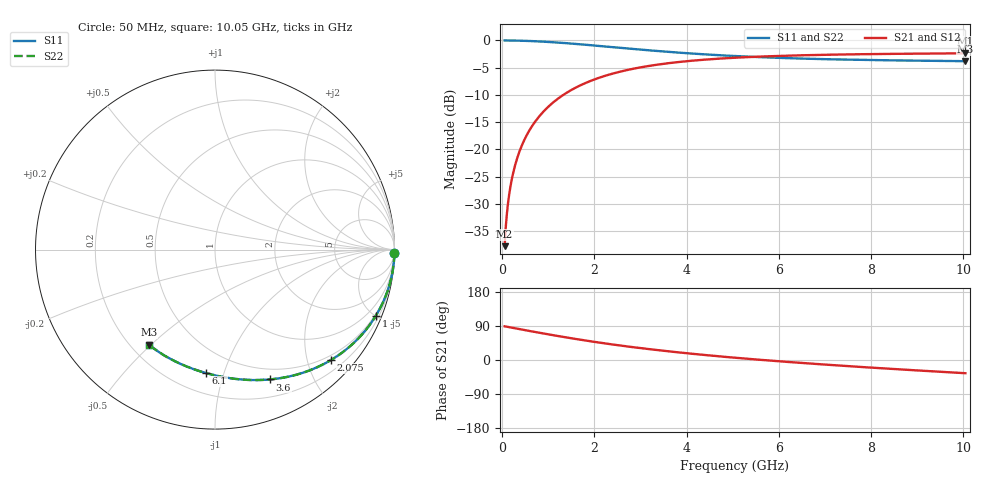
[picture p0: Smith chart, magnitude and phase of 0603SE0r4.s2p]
! AVX Thin Film Operation		Date: August 2001
! Description: Accu-P® Series, Thin Film, SMD, RF Capacitor
! Part Number: 06035J0R4ABT
! 50 MHz  -  10.05 GHz
! Serial Measurements
# mhz S db R 50
!	S11		S21		S12		S22
!	dB	Phase	dB	Phase	dB	Phase	dB	Phase
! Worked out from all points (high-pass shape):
!   401 points, 50 MHz to 10.05 GHz, reference 50 ohm
!   highest |S21| = -2.36 dB at 10.05 GHz (marker M1); lowest = -37.8 dB at 50 MHz (marker M2)
!   |S21| within 3 dB of the highest: 2.751 GHz to end of sweep
!   lowest |S11| = -3.8 dB at 10.05 GHz (marker M3), VSWR 4.64, Z = 13.6 - j24.6 ohm
!   |S11| at or under -10 dB: nowhere
!   |S22| runs from -3.8 to 0.0 dB; largest |S21 - S12| = 6.7e-05
!   S11 on the Smith chart (normalised r, x): 50 MHz: open; 1 GHz: 0.42, -5.02; 2.075 GHz: 0.41, -2.45; 3.6 GHz: 0.38, -1.44; 6.1 GHz: 0.33, -0.87; 10.05 GHz: 0.27, -0.49
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50  -0.00 -1.1  -37.79 88.9  -37.79 88.9  -0.00 -1.1
75  -0.00 -1.7  -34.27 88.3  -34.27 88.3  -0.00 -1.7
125  -0.00 -2.9  -29.84 87.1  -29.84 87.1  -0.00 -2.9
175  -0.01 -4.0  -26.92 86.0  -26.92 86.0  -0.01 -4.0
250  -0.02 -5.7  -23.84 84.3  -23.84 84.3  -0.02 -5.7
350  -0.04 -8.0  -20.94 82.0  -20.94 82.0  -0.04 -8.0
475  -0.07 -10.8  -18.33 79.2  -18.33 79.2  -0.07 -10.8
625  -0.11 -14.2  -16.01 75.8  -16.01 75.8  -0.11 -14.2
800  -0.18 -18.0  -13.96 72.0  -13.96 72.0  -0.18 -18.0
1000  -0.27 -22.4  -12.17 67.6  -12.17 67.6  -0.27 -22.4
1325  -0.46 -29.2  -10.00 60.8  -10.00 60.8  -0.46 -29.2
1725  -0.73 -37.1  -8.12 52.9  -8.12 52.9  -0.73 -37.1
2075  -0.99 -43.5  -6.93 46.5  -6.93 46.5  -0.99 -43.5
2675  -1.44 -53.6  -5.50 36.4  -5.50 36.4  -1.44 -53.6
3400  -1.96 -64.3  -4.41 25.7  -4.41 25.7  -1.96 -64.3
3600  -2.09 -67.0  -4.18 23.0  -4.18 23.0  -2.09 -67.0
4300  -2.51 -75.7  -3.59 14.3  -3.59 14.3  -2.50 -75.7
5050  -2.86 -83.9  -3.17 6.0  -3.17 6.0  -2.86 -83.9
6100  -3.23 -94.2  -2.81 -4.2  -2.81 -4.2  -3.23 -94.1
6725  -3.38 -99.7  -2.68 -9.7  -2.68 -9.7  -3.38 -99.6
8400  -3.65 -113.0  -2.47 -23.1  -2.47 -23.1  -3.65 -112.9
10050  -3.81 -124.8  -2.36 -34.9  -2.36 -34.9  -3.81 -124.7
